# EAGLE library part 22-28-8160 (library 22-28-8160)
Headers & Wire Housings BKWY HDR R/A 16P tin Source: Datasheet
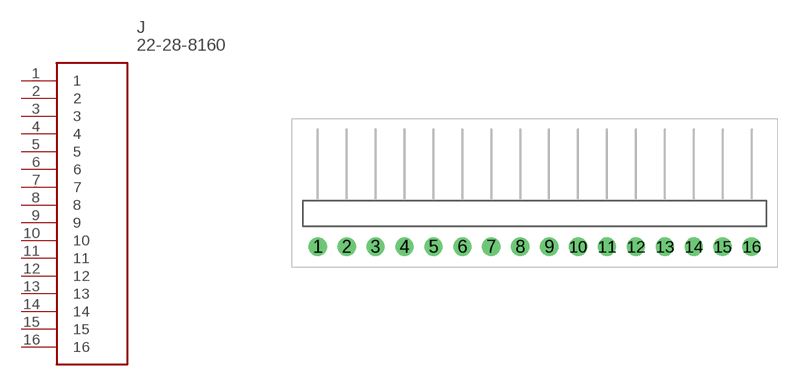
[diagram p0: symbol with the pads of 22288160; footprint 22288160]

Designator prefix J

## 22-28-8160 (Description: Headers & Wire Housings BKWY HDR R/A 16P tin; Height: 2mm; Manufacturer_Name: Molex; Manufacturer_Part_Number: 22-28-8160; Mouser_Part_Number: 538-22-28-8160; Mouser_Price-Stock: https://www.mouser.com/Search/Refine.aspx?Keyword=538-22-28-8160)  [22288160]
1  1
2  2
3  3
4  4
5  5
6  6
7  7
8  8
9  9
10  10
11  11
12  12
13  13
14  14
15  15
16  16

## Footprint 22288160 (pad centres in mm)
22-28-8160
drill 1.07 pad 1.605: 1 -19.05,-4.734; 2 -16.51,-4.734; 3 -13.97,-4.734; 4 -11.43,-4.734; 5 -8.89,-4.734; 6 -6.35,-4.734; 7 -3.81,-4.734; 8 -1.27,-4.734; 9 1.27,-4.734; 10 3.81,-4.734; 11 6.35,-4.734; 12 8.89,-4.734; 13 11.43,-4.734; 14 13.97,-4.734; 15 16.51,-4.734; 16 19.05,-4.734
